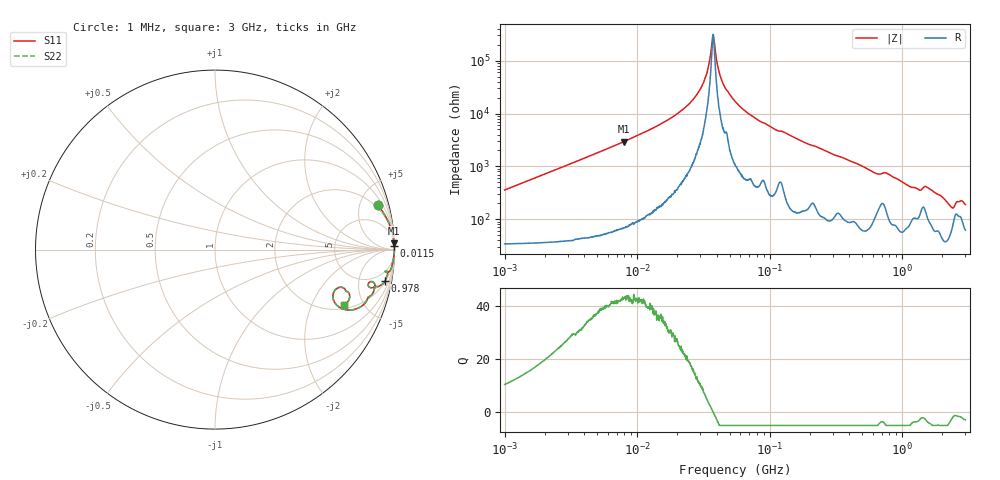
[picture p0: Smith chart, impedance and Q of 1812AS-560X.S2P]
!s-Parameter Generated by FASTRON Sdn. Bhd.
!FASTRON P/N : 1812AS-560X
!Keysight Technologies,E4991B,MY54100416,A.01.15
!Date created: Mon Oct 16 10:15:08 2023
!Version  : Rev00 Mon Oct 16 10:15:08 2023
!Data & Calibration Information:
!Freq	S11	S21	S12	S22
!PortZ  Port1:50+j0  Port2:50+j0
!When reading, reference impedance value at option line is always used.
! Remarks : This data is being provided solely for informational purposes.
# Hz S dB R 50
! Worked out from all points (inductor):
!   1601 points, 1 MHz to 3 GHz, reference 50 ohm
!   read as one part in series: L = 56.4 uH near 1.041 MHz
!   highest Q = 43.2 at 7.898 MHz (marker M1), where L = 58.8 uH
!   self-resonance near 37.45 MHz
!   S11 on the Smith chart (normalised r, x): 1 MHz: 1.68, +7.09; 11.5 MHz: 3, +89; 978 MHz: 2, -10; 3 GHz: 2.24, -3.57
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1000000  -0.54 15.2  -11.58 -69.3  -11.58 -69.3  -0.54 15.2
3804036  -0.04 4.2  -22.71 -84.0  -22.71 -84.0  -0.04 4.2
7898269  -0.01 2.0  -29.31 -86.7  -29.31 -86.7  -0.01 2.0
1.149534e7  -0.01 1.3  -33.02 -87.3  -33.02 -87.3  -0.01 1.3
1.447069e7  -0.01 1.0  -35.55 -87.4  -35.55 -87.4  -0.01 1.0
2.20312e7  -0.00 0.5  -41.45 -86.9  -41.45 -86.9  -0.00 0.5
2.87222e7  -0.00 0.2  -47.70 -84.9  -47.70 -84.9  -0.00 0.2
3.320783e7  -0.00 0.1  -54.53 -79.4  -54.53 -79.4  -0.00 0.1
3.74453e7  -0.00 0.0  -69.93 -5.1  -69.93 -5.1  -0.00 0.0
4.37287e7  -0.00 -0.1  -52.25 81.4  -52.25 81.4  -0.00 -0.1
5.477226e7  -0.00 -0.3  -44.63 86.0  -44.63 86.0  -0.00 -0.3
8.422788e7  -0.01 -0.8  -37.11 85.7  -37.11 85.7  -0.01 -0.8
2.083556e8  -0.03 -2.3  -27.96 83.2  -27.96 83.2  -0.03 -2.3
6.233561e8  -0.24 -7.4  -17.70 74.4  -17.70 74.4  -0.24 -7.4
7.925923e8  -0.25 -7.8  -17.21 74.1  -17.21 74.1  -0.25 -7.8
9.779672e8  -0.32 -10.5  -14.74 73.3  -14.74 73.3  -0.32 -10.5
1.333714e9  -0.94 -13.7  -12.09 59.0  -12.09 59.0  -0.94 -13.7
1.519029e9  -0.82 -12.2  -13.11 60.1  -13.11 60.1  -0.82 -12.2
2.000286e9  -1.02 -19.3  -9.48 61.3  -9.48 61.3  -1.02 -19.3
2.312676e9  -2.18 -24.9  -7.12 48.0  -7.12 48.0  -2.18 -24.9
2.568929e9  -2.54 -16.6  -8.99 36.8  -8.99 36.8  -2.54 -16.6
3e9  -2.12 -23.1  -7.63 47.8  -7.63 47.8  -2.12 -23.1
